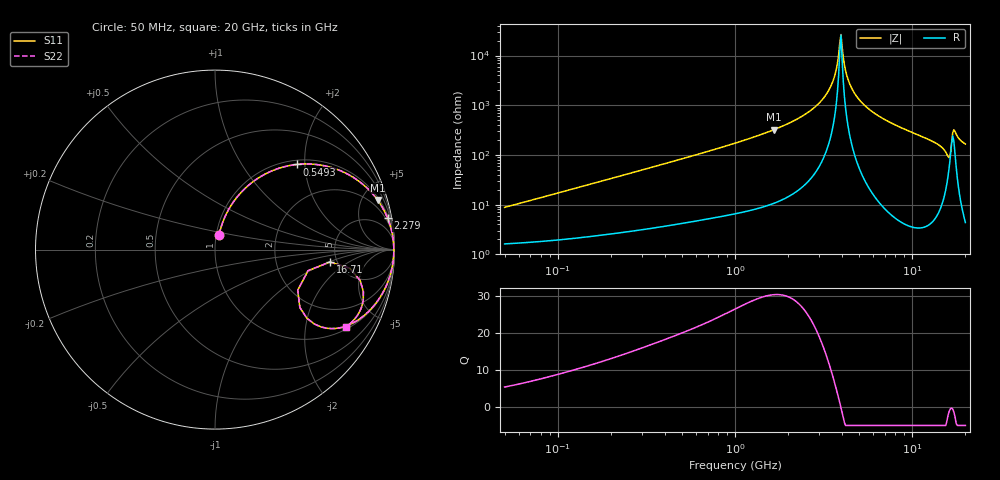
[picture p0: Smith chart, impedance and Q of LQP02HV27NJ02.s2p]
!Murata Part Number: LQP02HV27NJ02
!These Parameters are Measured in Series Mode Connection
!  o--[Z]--o
!Port1  Port2
!  o-------o
!Freq. Start=50[MHz] Stop=20[GHz], 401[Steps]
# Hz S RI R 50
!Freq.(Hz) S11(Real) S11(Imag) S21(Real) S21(Imag) S12(Real) S12(Imag) S22(Real) S22(Imag)
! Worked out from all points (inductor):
!   401 points, 50 MHz to 20 GHz, reference 50 ohm
!   read as one part in series: L = 27.4 nH near 51.52 MHz
!   highest Q = 30.2 at 1.664 GHz (marker M1), where L = 31 nH
!   self-resonance near 3.908 GHz
!   S11 on the Smith chart (normalised r, x): 50 MHz: 1.03, +0.17; 549.3 MHz: 1.09, +1.83; 2.279 GHz: 1, +11; 16.71 GHz: 4.37, -1.03; 20 GHz: 1.09, -3.32
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5e7  0.0231 0.0834  0.9769 -0.0834  0.9769 -0.0834  0.0231 0.0834
1.364002e8  0.069 0.2105  0.931 -0.2105  0.931 -0.2105  0.069 0.2105
3.721004e8  0.2883 0.4254  0.7117 -0.4254  0.7117 -0.4254  0.2883 0.4254
5.492803e8  0.4581 0.4746  0.5419 -0.4746  0.5419 -0.4746  0.4581 0.4746
1e9  0.7404 0.4198  0.2596 -0.4198  0.2596 -0.4198  0.7404 0.4198
1.664083e9  0.9055 0.2765  0.0945 -0.2765  0.0945 -0.2765  0.9055 0.2765
2.279204e9  0.9616 0.1752  0.0384 -0.1752  0.0384 -0.1752  0.9616 0.1752
2.728004e9  0.9807 0.1175  0.0193 -0.1175  0.0193 -0.1175  0.9807 0.1175
3.466789e9  0.9942 0.0417  0.00584 -0.0417  0.00584 -0.0417  0.9942 0.0417
3.680849e9  0.9956 0.0228  0.00441 -0.0228  0.00441 -0.0228  0.9956 0.0228
3.850025e9  0.9962 0.00865  0.00383 -0.00865  0.00383 -0.00865  0.9962 0.00865
3.967106e9  0.9963 -0.000791  0.00367 0.000791  0.00367 0.000791  0.9963 -0.000791
4.34015e9  0.9957 -0.0292  0.00431 0.0292  0.00431 0.0292  0.9957 -0.0292
4.748272e9  0.9934 -0.0578  0.00665 0.0578  0.00665 0.0578  0.9934 -0.0578
5.683258e9  0.9833 -0.1159  0.0167 0.1159  0.0167 0.1159  0.9833 -0.1159
7.442007e9  0.9521 -0.2064  0.0479 0.2064  0.0479 0.2064  0.9521 -0.2064
1.183995e10  0.8255 -0.3716  0.1745 0.3716  0.1745 0.3716  0.8255 -0.3716
1.482269e10  0.649 -0.4401  0.351 0.4401  0.351 0.4401  0.649 -0.4401
1.597544e10  0.4727 -0.3225  0.5273 0.3225  0.5273 0.3225  0.4727 -0.3225
1.670968e10  0.6406 -0.069  0.3594 0.069  0.3594 0.069  0.6406 -0.069
1.774144e10  0.8259 -0.2834  0.1741 0.2834  0.1741 0.2834  0.8259 -0.2834
2e10  0.7281 -0.4319  0.2719 0.4319  0.2719 0.4319  0.7281 -0.4319
